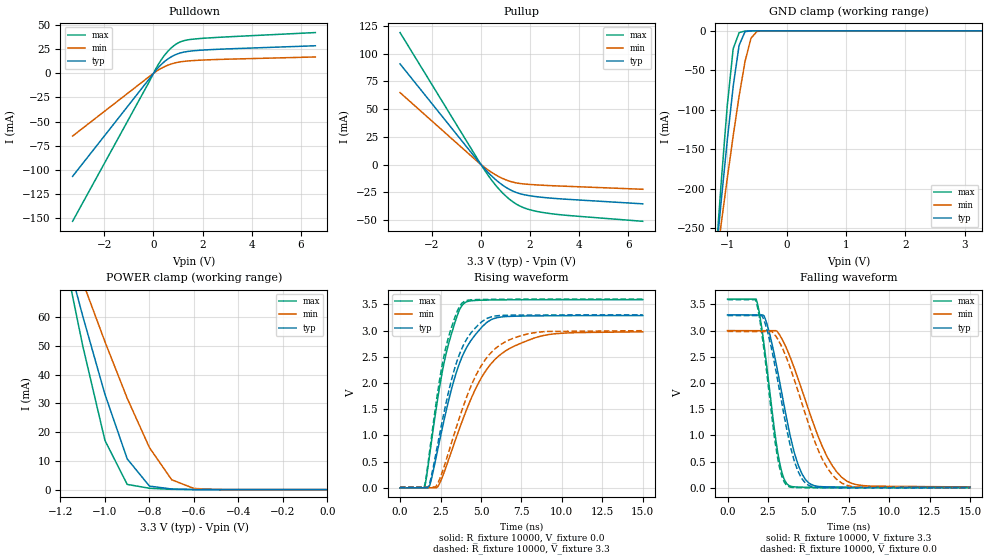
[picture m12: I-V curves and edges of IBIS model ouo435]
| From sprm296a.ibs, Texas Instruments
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[Model]   ouo435
Model_type   3-state
Enable   Active-Low
Polarity   Non-Inverting
| signals   A, GZ, Y
Vmeas = 1.5
|   typ   min   max
C_comp   2.5478p   2.5389p   2.6979p
|   typ   min   max
[Temperature Range]   25   -40   125
|   typ   min   max
[Voltage Range]   3.30V   3.00V   3.60V
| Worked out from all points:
|   slope of the pulldown table from 0 to 0.495 V, typ, clamps not added: 37.7 ohm
|   slope of the pullup table from 0 to 0.495 V, typ, clamps not added: 42.7 ohm
|   GND clamp passes 1 mA (typ) near -0.69 V on its own axis
|   POWER clamp passes 1 mA (typ) near -0.78 V on its own axis
|   rising waveform, R_fixture 10000, V_fixture 0.0: 20-80 % time 1.75ns typ, 2.6ns min, 1.25ns max; typ from 0 V to 3.29 V
|   falling waveform, R_fixture 10000, V_fixture 3.3: 20-80 % time 1.31ns typ, 2.14ns min, 884ps max; typ from 3.3 V to 0.01 V
|   rising waveform, R_fixture 10000, V_fixture 3.3: 20-80 % time 1.58ns typ, 2.24ns min, 1.16ns max; typ from 0.01 V to 3.3 V
|   falling waveform, R_fixture 10000, V_fixture 0.0: 20-80 % time 1.26ns typ, 2.03ns min, 865ps max; typ from 3.29 V to 0 V
[Pulldown]
|   Voltage   I(typ)   I(min)   I(max)
-3.3V     -106.6mA   -64.91mA   -153.1mA
-200mV    -6.638mA   -3.888mA   -9.861mA
200mV     6.136mA    3.487mA    9.379mA
500mV     13.23mA    7.514mA    20.3mA
800mV     18.12mA    10.25mA    27.98mA
1V        20.32mA    11.45mA    31.43mA
1.2V      21.76mA    12.24mA    33.52mA
1.7V      23.5mA     13.33mA    35.59mA
6.6V      28.52mA    16.93mA    42.18mA
[GND_clamp]
|   Voltage   I(typ)   I(min)   I(max)
-3.3V     -2.08A     -1.591A    -2.668A
-1.2V     -293.5mA   -301.6mA   -294.1mA
-1.1V     -214.7mA   -243.9mA   -190.7mA
-1V       -139.3mA   -187.5mA   -95.2mA
-900mV    -70.62mA   -133.4mA   -22.79mA
-800mV    -18.33mA   -82.78mA   -2.33mA
-700mV    -1.069mA   -38.92mA   -224.2uA
-600mV    -42.87uA   -9.385mA   -12.72uA
-500mV    -2.084uA   -800.4uA   -442.1nA
-300mV    -3.891nA   -2.62uA    -449.6pA
3.3V      222pA      359nA      177.6pA
[Pullup]
|   Voltage   I(typ)   I(min)   I(max)
-3.3V     90.83mA    64.92mA    119.1mA
100mV     -2.569mA   -1.78mA    -3.482mA
400mV     -9.588mA   -6.59mA    -13.07mA
700mV     -15.54mA   -10.57mA   -21.33mA
1.2V      -22.92mA   -15.27mA   -32mA
1.7V      -26.98mA   -17.44mA   -38.62mA
2V        -28.23mA   -18.01mA   -40.89mA
2.5V      -29.63mA   -18.7mA    -43.25mA
3.5V      -31.38mA   -19.67mA   -45.9mA
6.6V      -35.51mA   -22.36mA   -51.28mA
[POWER_clamp]
|   Voltage   I(typ)   I(min)   I(max)
-3.3V     758.3mA    581mA      973mA
-1.2V     89.56mA    93.92mA    87.99mA
-1.1V     60.47mA    72.37mA    50.13mA
-1V       33.18mA    51.49mA    17.12mA
-900mV    10.7mA     31.81mA    1.812mA
-800mV    1.221mA    14.62mA    465.8uA
-700mV    206.6uA    3.422mA    95.32uA
-600mV    31.41uA    399uA      7.822uA
-500mV    2.639uA    43.56uA    300.6nA
0V        1pA        1pA        1pA
[Ramp]
|   I(typ)   I(min)   I(max)
dV/dt_r   1.972/1.746n   1.786/2.595n   2.154/1.244n
dV/dt_f   1.974/1.304n   1.790/2.139n   2.156/0.880n
[Rising Waveform]
R_fixture = 10000
V_fixture = 0.0
|  pu_on
|  TIME   V(typ)   V(min)   V(max)
0s        5nV        13nV       4nV
1.527ns   788.1uV    1.015mV    14.27mV
1.833ns   43.4mV     1.015mV    639.7mV
2.343ns   749.1mV    24.15mV    1.73V
2.751ns   1.334V     318.8mV    2.43V
3.465ns   2.189V     951.5mV    3.223V
3.975ns   2.593V     1.382V     3.526V
5.3ns     3.139V     2.235V     3.582V
7.034ns   3.273V     2.699V     3.588V
15ns      3.287V     2.977V     3.59V
[Falling Waveform]
R_fixture = 10000
V_fixture = 3.3
V_fixture_min = 3.0
V_fixture_max = 3.6
|  pd_on
|  TIME   V(typ)   V(min)   V(max)
0s        3.3V       3V         3.6V
1.771ns   3.298V     2.998V     3.6V
2.34ns    3.216V     2.998V     2.534V
3.153ns   2.135V     2.949V     588mV
3.804ns   1.098V     2.546V     42.79mV
4.373ns   432.7mV    2.069V     15.36mV
4.86ns    142.8mV    1.627V     11.45mV
6.161ns   18.97mV    590.9mV    8.214mV
7.299ns   13.93mV    144.9mV    7.506mV
15ns      9.873mV    17.28mV    6.999mV
[Rising Waveform]
R_fixture = 10000
V_fixture = 3.3
V_fixture_min = 3.0
V_fixture_max = 3.6
|  pd_off
|  TIME   V(typ)   V(min)   V(max)
0s        9.792mV    15.69mV    6.993mV
1.485ns   10.55mV    16.73mV    6.993mV
1.808ns   63.27mV    16.73mV    651.8mV
2.213ns   650.1mV    26.35mV    1.586V
2.698ns   1.408V     382.6mV    2.493V
3.264ns   2.159V     943.9mV    3.139V
3.83ns    2.664V     1.484V     3.524V
5.205ns   3.2V       2.417V     3.594V
6.742ns   3.293V     2.821V     3.598V
15ns      3.3V       2.998V     3.6V
[Falling Waveform]
R_fixture = 10000
V_fixture = 0.0
|  pu_off
|  TIME   V(typ)   V(min)   V(max)
0s        3.287V     2.984V     3.59V
1.766ns   3.285V     2.982V     3.561V
2.317ns   3.142V     2.982V     2.474V
3.075ns   2.094V     2.851V     608.7mV
3.696ns   1.064V     2.439V     40.6mV
4.178ns   467.1mV    2.015V     6.069mV
4.798ns   96.84mV    1.42V      2.342mV
5.901ns   3.471mV    523.6mV    637.3uV
7.004ns   1.37mV     104.2mV    266.9uV
15ns      23.56uV    282uV      4.151uV
